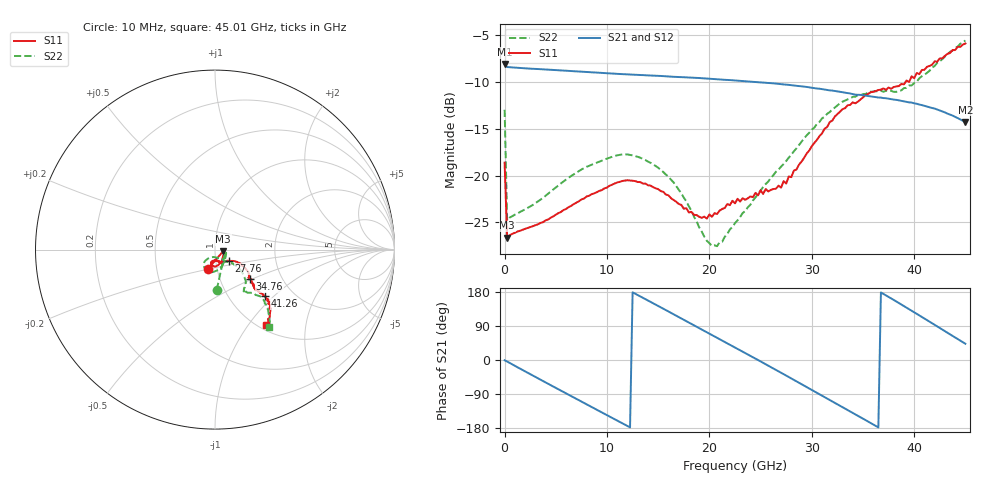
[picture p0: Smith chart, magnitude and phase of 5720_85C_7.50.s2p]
! Device:  ADRF5720
! Description: 0.5dB LSB GaAs MMIC 6-bit Digital Attenuator
! Frequency:  0.000009 -  40 GHz
! Ports:
!	RF1	= Port 1
!	RF2	= Port 2
! Vdd:  3.3 Volt
! Vss:  -3.3 Volt
! Control:  0/3.3 Volt
! State:  7.50 dB attenuation
! Data:  The device was measured using G-S-G Probes on a matrix board.
!  Data was collected using an calibrated 4 port network analyzer.
!  The reference plane for this measurement is at the launchers.
! Note:  Analog Devices supplies this data as a sample of measured data
!  for this product.  Your particular data for this product may vary.
!  Data was taken at 85 degrees C.
!  Analog Devices reserves the right to change this data at anytime.
# GHZ S DB R 45.0
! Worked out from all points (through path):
!   181 points, 10 MHz to 45.01 GHz, reference 45 ohm
!   highest |S21| = -8.11 dB at 10 MHz (marker M1); lowest = -14.3 dB at 45.01 GHz (marker M2)
!   group delay of S21, straight-line fit = 41.3 ps
!   lowest |S11| = -26.6 dB at 260 MHz (marker M3), VSWR 1.10, Z = 49.3 - j0.842 ohm
!   |S11| at or under -10 dB: start of sweep to 39.16 GHz; 39.49529 GHz to 39.5141 GHz (18.8 MHz wide, 0.0476 % of centre)
!   |S22| runs from -27.5 to -5.6 dB; largest |S21 - S12| = 0.0019
!   S11 on the Smith chart (normalised r, x): 10 MHz: 0.90, -0.20; 27.76 GHz: 1.16, -0.15; 34.76 GHz: 1.39, -0.49; 41.26 GHz: 1.46, -0.88; 45.01 GHz: 1.08, -1.22
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0.01  -18.62 -110.5  -8.11 -0.8  -8.09 -0.8  -12.97 -87.6
0.26  -26.63 -10.5  -8.41 -4.0  -8.40 -4.0  -24.75 -8.9
2.26  -25.59 -18.4  -8.56 -33.7  -8.54 -33.6  -23.44 -23.6
4.26  -24.68 -39.2  -8.68 -62.8  -8.67 -62.7  -21.93 -48.0
6.01  -23.56 -51.2  -8.80 -88.1  -8.78 -88.0  -20.42 -63.3
7.76  -22.45 -61.6  -8.92 -113.3  -8.90 -113.2  -19.21 -76.0
11.51  -20.57 -86.4  -9.16 -167.1  -9.15 -166.9  -17.74 -102.5
13.26  -20.69 -96.8  -9.26 167.8  -9.25 168.0  -18.09 -113.6
15.26  -21.65 -105.1  -9.36 138.9  -9.35 139.1  -19.39 -125.1
17.76  -23.48 -103.0  -9.51 102.7  -9.50 102.9  -22.76 -130.2
20.26  -24.39 -83.0  -9.67 66.2  -9.65 66.4  -27.50 -100.9
21.26  -23.56 -77.0  -9.75 51.5  -9.73 51.7  -27.06 -80.5
22.76  -22.47 -68.7  -9.86 29.5  -9.85 29.7  -24.77 -60.7
25.26  -21.95 -60.7  -10.07 -7.4  -10.05 -7.2  -21.20 -47.9
27.01  -21.28 -46.9  -10.23 -33.6  -10.22 -33.4  -19.04 -40.0
27.76  -20.09 -39.3  -10.31 -44.9  -10.30 -44.6  -18.08 -38.8
30.26  -16.51 -30.4  -10.66 -82.7  -10.64 -82.5  -14.87 -38.7
32.26  -13.69 -32.5  -10.96 -113.0  -10.94 -112.7  -12.74 -44.0
34.76  -11.87 -39.9  -11.38 -150.9  -11.37 -150.6  -11.45 -52.5
37.76  -10.73 -43.0  -11.84 162.4  -11.82 162.8  -10.95 -54.6
41.26  -8.38 -42.6  -12.62 105.2  -12.60 105.6  -9.02 -46.6
45.01  -5.89 -55.9  -14.28 42.9  -14.25 43.2  -5.57 -55.0
